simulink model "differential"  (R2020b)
settings: Solver=FixedStepAuto  StartTime=0.0  StopTime=10  FixedStep=0.02  RelTol=1e-3
libraries: sldrtlib x1

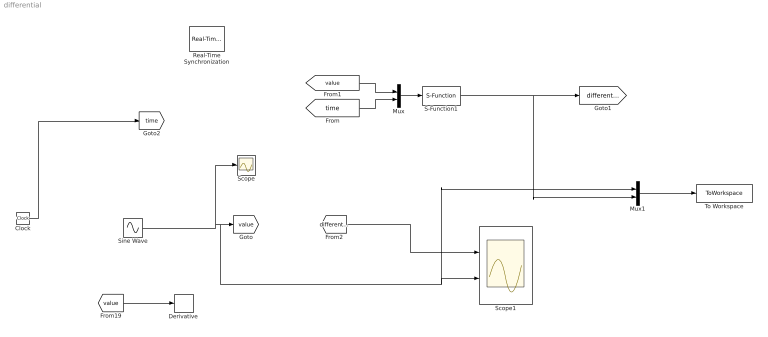
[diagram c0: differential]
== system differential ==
  Clock : Clock
  Derivative : Derivative
  Mux : Mux  Inputs=2
  Mux1 : Mux  Inputs=2
  Real-Time Synchronization : sldrtlib/Real-Time Synchronization  SampleTime=0.02  MaxMissedTicks=inf  ShowMissedTicks=off  YieldWhenWaiting=off
  S-Function1 : S-Function  FunctionName=modbusComdiff  SFunctionDeploymentMode=off  EnableBusSupport=off
  Scope : Scope
  Scope1 : Scope  NumInputPorts=2
  Sine Wave : Sin  Amplitude=10  SampleTime=0
  To Workspace : ToWorkspace  VariableName=simout  SampleTime=-1
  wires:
  [value] -> Derivative/1
  [value] -> Mux/1
  [time] -> Mux/2
  Mux/1 -> S-Function1/1
  Clock/1 -> [time]
  [differential] -> Scope1/1
  Mux1/1 -> To Workspace/1
  Sine Wave/1 -> Scope/1, Mux1/1, Scope1/2, [value]
  S-Function1/1 -> Mux1/2, [differential]
